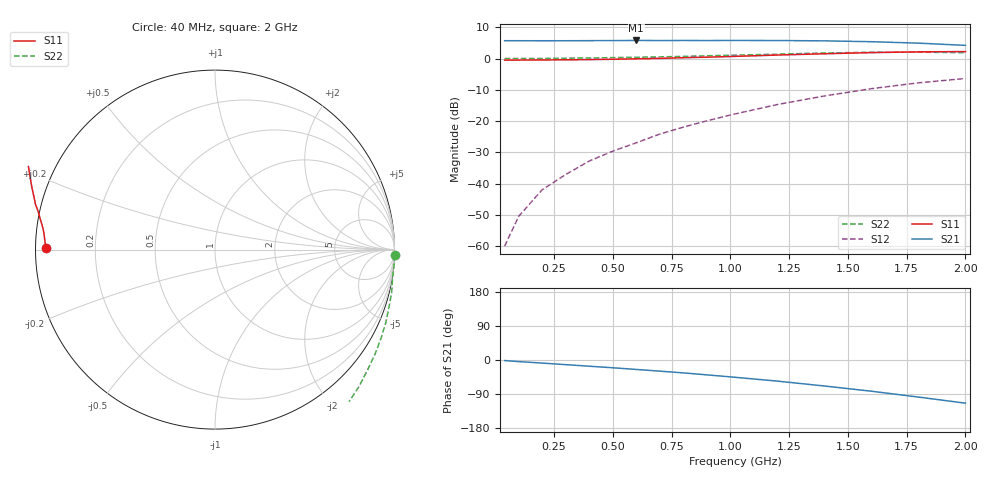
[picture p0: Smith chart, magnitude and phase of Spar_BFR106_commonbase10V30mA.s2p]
! Filename:  BFR106CF.S2P  Version:  2.0
! NXP part #: BFR106  Date: Jul 1990
! Bias condition: Vce=10V, Ic=30mA
! COMMON BASE
#  MHz  S  MA  R  50
! Freq  S11  S21  S12  S22
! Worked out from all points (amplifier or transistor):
!   16 points, 40 MHz to 2 GHz, reference 50 ohm
!   highest |S21| = 5.8 dB at 600 MHz (marker M1)
!   |S21| within 3 dB of that: start of sweep to end of sweep
!   unconditionally stable (mu >= 1): nowhere
!   at 200 MHz: K = -0.49, MSG = 23.8 dB, |S12| = -41.9 dB
!   at 800 MHz: K = -0.91, MSG = 13.9 dB, |S12| = -21.9 dB
!   at 2 GHz: K = -0.80, MSG = 5.3 dB, |S12| = -6.4 dB
40  0.944 179.5  1.929 -1.5  0.001 58.3  1.001 -1.8
100  0.946 178.1  1.928 -4.2  0.003 97.3  1.002 -4.5
200  0.95 176.8  1.926 -8.1  0.008 116.5  1.002 -9.0
300  0.955 175.2  1.927 -12.3  0.014 129.4  1.013 -13.8
400  0.963 173.4  1.933 -16.4  0.023 134.5  1.021 -18.3
500  0.974 171.8  1.937 -20.5  0.033 136.5  1.035 -23.2
600  0.99 169.9  1.947 -24.9  0.045 138.1  1.048 -27.9
700  1.007 167.9  1.941 -29.4  0.062 138.7  1.064 -32.9
800  1.032 165.8  1.945 -34.0  0.08 138.4  1.082 -38.1
900  1.052 163.6  1.942 -39.2  0.101 137.0  1.107 -43.5
1000  1.078 161.2  1.946 -44.5  0.125 135.1  1.129 -48.6
1200  1.138 156.0  1.942 -55.7  0.184 129.9  1.174 -60.3
1400  1.193 149.5  1.919 -68.6  0.252 123.2  1.228 -72.5
1600  1.245 142.0  1.859 -82.4  0.33 115.7  1.259 -85.9
1800  1.28 133.8  1.763 -97.8  0.409 106.5  1.264 -100.1
2000  1.292 125.7  1.625 -113.9  0.48 97.4  1.243 -114.7
